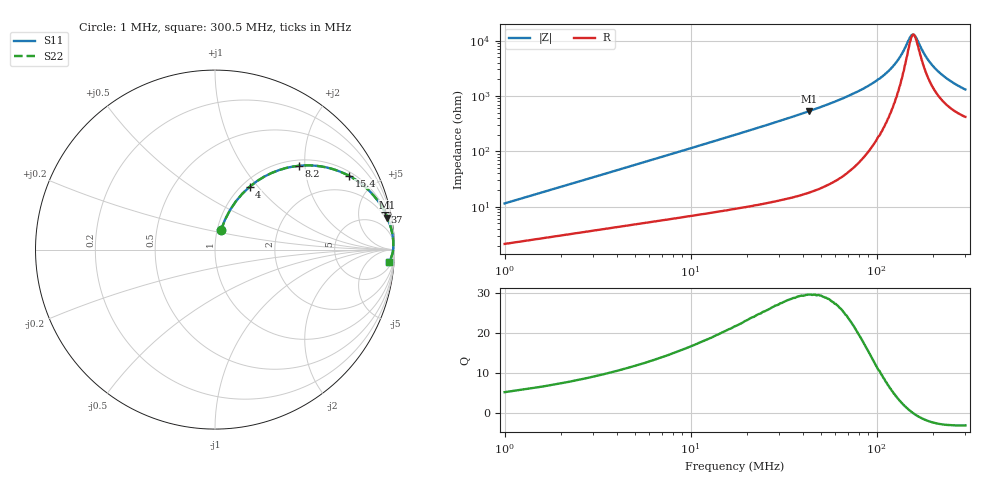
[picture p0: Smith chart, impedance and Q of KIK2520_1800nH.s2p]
!version-2
!date-01.2022
!Series
# MHz S RI R 50
!Freq ReS11 ImS11 ReS21 ImS21 ReS12 ImS12 ReS22 ImS22
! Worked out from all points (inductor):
!   500 points, 1 MHz to 300.5 MHz, reference 50 ohm
!   read as one part in series: L = 1.8 uH near 2.2 MHz
!   highest Q = 29.5 at 43.6 MHz (marker M1), where L = 1.95 uH
!   self-resonance near 158.5 MHz
!   S11 on the Smith chart (normalised r, x): 1 MHz: 1.04, +0.23; 4 MHz: 1.09, +0.91; 8.2 MHz: 1.12, +1.86; 15.4 MHz: 1.17, +3.52; 37 MHz: 1.31, +8.86; 300.5 MHz: 9, -25
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1  0.0328 0.1071  0.9672 -0.1071  0.9672 -0.1071  0.0328 0.1071
2.8  0.1172 0.27  0.8828 -0.27  0.8828 -0.27  0.1172 0.27
4  0.1931 0.3502  0.8069 -0.3502  0.8069 -0.3502  0.1931 0.3502
5.8  0.316 0.4272  0.684 -0.4272  0.684 -0.4272  0.316 0.4272
8.2  0.467 0.4669  0.533 -0.4669  0.533 -0.4669  0.467 0.4669
11.8  0.6365 0.4541  0.3635 -0.4541  0.3635 -0.4541  0.6365 0.4541
15.4  0.7458 0.4117  0.2542 -0.4117  0.2542 -0.4117  0.7458 0.4117
23.8  0.8741 0.3122  0.1259 -0.3122  0.1259 -0.3122  0.8741 0.3122
37  0.9449 0.2114  0.0551 -0.2114  0.0551 -0.2114  0.9449 0.2114
43.6  0.9605 0.1785  0.0395 -0.1785  0.0395 -0.1785  0.9605 0.1785
51.4  0.9721 0.1484  0.0279 -0.1484  0.0279 -0.1484  0.9721 0.1484
101  0.9929 0.0507  0.00709 -0.0507  0.00709 -0.0507  0.9929 0.0507
128  0.9937 0.0237  0.00626 -0.0237  0.00626 -0.0237  0.9937 0.0237
140  0.9934 0.0136  0.00662 -0.0136  0.00662 -0.0136  0.9934 0.0136
151  0.9927 0.00503  0.00725 -0.00503  0.00725 -0.00503  0.9927 0.00503
156.5  0.9924 0.00121  0.00764 -0.00121  0.00764 -0.00121  0.9924 0.00121
161  0.992 -0.00166  0.00796 0.00166  0.00796 0.00166  0.992 -0.00166
181  0.9901 -0.0145  0.00992 0.0145  0.00992 0.0145  0.9901 -0.0145
201  0.9877 -0.0256  0.0123 0.0256  0.0123 0.0256  0.9877 -0.0256
223  0.9846 -0.0369  0.0154 0.0369  0.0154 0.0369  0.9846 -0.0369
251  0.9802 -0.0494  0.0198 0.0494  0.0198 0.0494  0.9802 -0.0494
300.5  0.9712 -0.0687  0.0288 0.0687  0.0288 0.0687  0.9712 -0.0686
